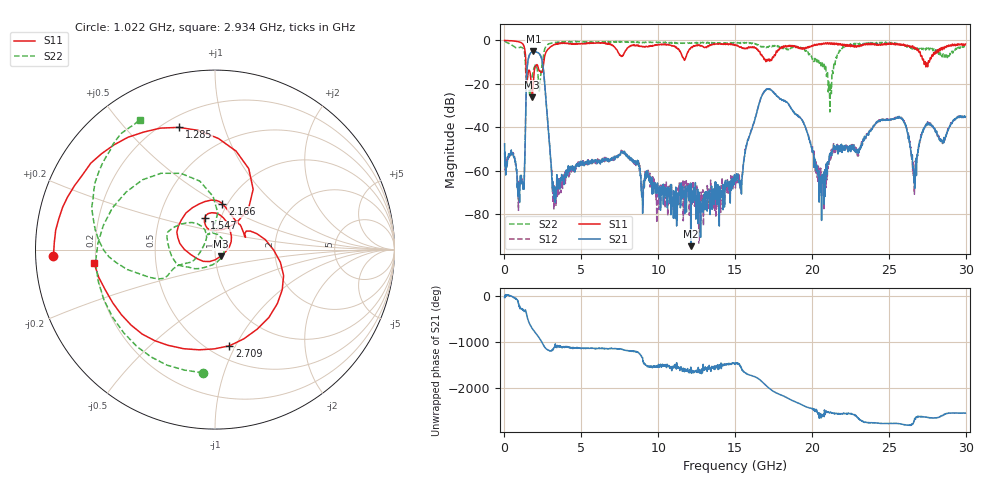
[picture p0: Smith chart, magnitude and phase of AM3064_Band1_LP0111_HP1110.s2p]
# Hz S DB R 50.0
!freq dBS11 angS11 dBS21 angS21 dBS12 angS12 dBS22 angS22
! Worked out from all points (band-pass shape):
!   1600 points, 10 MHz to 29.98 GHz, reference 50 ohm
!   highest |S21| = -5.06 dB at 1.884 GHz (marker M1); lowest = -94.8 dB at 12.12 GHz (marker M2)
!   |S21| within 3 dB of the highest: 1.568 GHz to 2.401 GHz (832.6 MHz wide, 42 % of centre)
!   lowest |S11| = -26.2 dB at 1.809 GHz (marker M3), VSWR 1.10, Z = 53.2 - j3.92 ohm
!   |S11| at or under -10 dB: 1.392 GHz to 2.554 GHz (1.162 GHz wide, 58.9 % of centre); 27.28038 GHz to 27.34913 GHz (68.74 MHz wide, 0.252 % of centre); 27.37 GHz to 27.57 GHz (203.9 MHz wide, 0.742 % of centre)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
!   |S22| runs from -33.0 to -0.4 dB; largest |S21 - S12| = 0.0074
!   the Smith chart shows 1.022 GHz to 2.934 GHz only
!   S11 on the Smith chart (normalised r, x): 1.022 GHz: 0.05, -0.02; 1.285 GHz: 0.26, +0.71; 1.547 GHz: 0.84, +0.30; 2.166 GHz: 0.95, +0.52; 2.709 GHz: 0.62, -0.95; 2.934 GHz: 0.19, -0.05
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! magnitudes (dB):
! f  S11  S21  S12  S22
! 10 MHz  -0.1  -47.7  -51.8  -0.4
! 1.022 GHz  -0.9  -66.5  -65.3  -3.2
! 1.285 GHz  -3.0  -63.8  -66.9  -5.0
! 1.547 GHz  -14.7  -8.7  -8.6  -20.4
! 1.809 GHz  -26.2  -5.2  -5.1  -16.3
! 1.884 GHz  -19.0  -5.1  -5.1  -13.7
! 2.166 GHz  -11.8  -5.6  -5.6  -15.1
! 2.709 GHz  -5.3  -28.2  -28.2  -2.7
! 2.934 GHz  -3.4  -47.7  -48.5  -1.6
! 3.271 GHz  -1.9  -67.4  -71.1  -1.0
! 5.015 GHz  -1.5  -56.6  -55.9  -0.6
! 10 GHz  -2.1  -70.0  -68.8  -1.0
! 12.12 GHz  -3.4  -94.8  -74.7  -1.3
! 15 GHz  -2.3  -64.9  -64.9  -1.3
! 17.07 GHz  -9.0  -22.5  -22.5  -3.1
! 19.99 GHz  -2.9  -49.8  -49.9  -8.1
! 20.74 GHz  -1.5  -63.1  -71.1  -11.5
! 25 GHz  -1.3  -36.6  -36.5  -1.2
! 25.97 GHz  -1.9  -37.3  -37.7  -2.6
! 26.68 GHz  -3.2  -68.3  -63.8  -4.1
! 27.45 GHz  -11.1  -39.3  -39.1  -3.6
! 29.98 GHz  -1.7  -35.2  -35.6  -3.0
